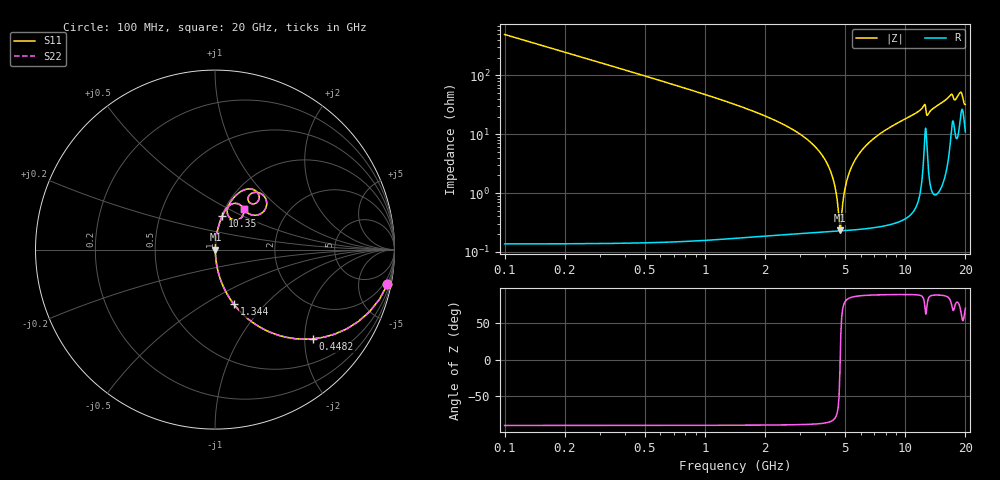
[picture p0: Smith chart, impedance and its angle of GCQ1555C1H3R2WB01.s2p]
!Murata Part Number: GCQ1555C1H3R2WB01
!These Parameters are Measured in Series Mode Connection
!Data Generated on Jan 08, 2026
!  o--ll--o
!Port1  Port2
!  o------o
!Operation Temp=25[degC], DC Bias Voltage=0[V]
!Freq. Start=100[MHz] Stop=20[GHz] 401[Steps]
# Hz S RI R 50
!Freq.(Hz) S11(Real) S11(Imag) S21(Real) S21(Imag) S12(Real) S12(Imag) S22(Real) S22(Imag)
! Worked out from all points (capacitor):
!   401 points, 100 MHz to 20 GHz, reference 50 ohm
!   read as one part in series: C = 3.2 pF near 199.5 MHz
!   lowest |Z| = 234 mohm at 4.727 GHz (marker M1)
!   series resonance near 4.74 GHz, so ESL is about 350 pH
!   S11 on the Smith chart (normalised r, x): 100 MHz: 1.00, -9.94; 448.2 MHz: 1.00, -2.20; 1.344 GHz: 1.00, -0.68; 10.35 GHz: 1.01, +0.39; 20 GHz: 1.22, +0.60
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1e8  0.9611 -0.1933  0.0389 0.1933  0.0389 0.1933  0.9611 -0.1933
4.4825e8  0.5472 -0.4971  0.4528 0.4971  0.4528 0.4971  0.5472 -0.4971
8.4625e8  0.2451 -0.4288  0.7549 0.4288  0.7549 0.4288  0.2451 -0.4288
1.34375e9  0.105 -0.3041  0.895 0.3041  0.895 0.3041  0.105 -0.3041
3.43325e9  0.00682 -0.0684  0.9932 0.0684  0.9932 0.0684  0.00682 -0.0684
4.279e9  0.00267 -0.0215  0.9973 0.0215  0.9973 0.0215  0.00267 -0.0215
4.478e9  0.00237 -0.012  0.9976 0.012  0.9976 0.012  0.00237 -0.012
4.72675e9  0.00226 -0.000599  0.9977 0.000599  0.9977 0.000599  0.00226 -0.000599
4.82625e9  0.00228 0.00378  0.9977 -0.00378  0.9977 -0.00378  0.00228 0.00378
5.075e9  0.00251 0.0144  0.9975 -0.0144  0.9975 -0.0144  0.00251 0.0144
5.3735e9  0.00304 0.0265  0.997 -0.0265  0.997 -0.0265  0.00304 0.0265
5.92075e9  0.00466 0.0473  0.9953 -0.0473  0.9953 -0.0473  0.00466 0.0473
6.7665e9  0.00849 0.0768  0.9915 -0.0768  0.9915 -0.0768  0.00849 0.0768
1.005e10  0.0359 0.1764  0.9641 -0.1764  0.9641 -0.1764  0.0359 0.1764
1.03485e10  0.0396 0.1851  0.9604 -0.1851  0.9604 -0.1851  0.0396 0.1851
1.2438e10  0.1251 0.2563  0.8749 -0.2563  0.8749 -0.2563  0.1251 0.2563
1.2836e10  0.095 0.1688  0.905 -0.1688  0.905 -0.1688  0.095 0.1688
1.338325e10  0.0695 0.2292  0.9305 -0.2292  0.9305 -0.2292  0.0695 0.2292
1.67165e10  0.199 0.3378  0.801 -0.3378  0.801 -0.3378  0.199 0.3378
1.7612e10  0.1967 0.2589  0.8033 -0.2589  0.8033 -0.2589  0.1967 0.2589
1.91045e10  0.288 0.2537  0.712 -0.2537  0.712 -0.2537  0.288 0.2537
2e10  0.1608 0.2276  0.8392 -0.2276  0.8392 -0.2276  0.1608 0.2276
